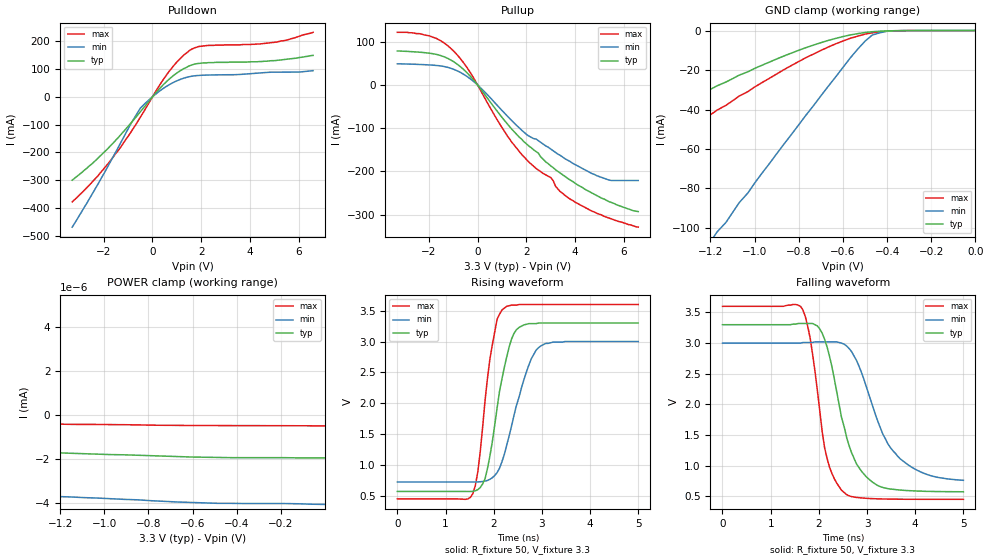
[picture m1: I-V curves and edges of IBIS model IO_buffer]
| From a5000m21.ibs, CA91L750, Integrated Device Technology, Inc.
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|   Model data
[Model]   IO_buffer
Model_type   I/O
Polarity   Non-Inverting
Enable   Active-Low
Vinl =   1.33V
Vinh =   1.74V
C_comp   5.0000pF   4.5000pF   5.5000pF
Rref = 0
Cref = 10pF
Vref = 2.0V
Vmeas = 0
|   |   |\ |   Rref
|   |Driver| \|------o----/\/\/\----o Vref
|   |   | /|   |
|   |   |/ |   === Cref
|   GND
[Temperature Range]   25.0000   80.0000   -40.0000
[Voltage Range]   3.3000V   3.0000V   3.6000V
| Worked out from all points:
|   slope of the pulldown table from 0 to 0.495 V, typ, clamps not added: 10.3 ohm
|   slope of the pullup table from 0 to 0.495 V, typ, clamps not added: 13.2 ohm
|   GND clamp passes 1 mA (typ) near -0.50 V on its own axis
|   POWER clamp passes 1 mA (typ) near -3.79 V on its own axis
|   rising waveform, R_fixture 50, V_fixture 3.3: 20-80 % time 357ps typ, 473ps min, 277ps max; typ from 0.571 V to 3.3 V
|   falling waveform, R_fixture 50, V_fixture 3.3: 20-80 % time 500ps typ, 711ps min, 343ps max; typ from 3.3 V to 0.573 V
[Pulldown]
|   voltage   I(typ)   I(min)   I(max)
-3.3V     -300mA     -469mA     -378mA
-2.5V     -242mA     -353mA     -309mA
-1.8V     -183mA     -245mA     -238mA
-1.3V     -136mA     -164mA     -180mA
-500mV    -54mA      -40.9mA    -73.6mA
500mV     48.4mA     33.5mA     69.2mA
900mV     79mA       53.5mA     115mA
1.3V      102mA      67.4mA     151mA
1.6V      114mA      73.8mA     171mA
1.9V      120mA      76.8mA     181mA
5.1V      131mA      88.7mA     197mA
6.6V      149mA      94.1mA     232mA
[Pullup]
|   voltage   I(typ)   I(min)   I(max)
-3.3V     78.9mA     49.1mA     122mA
-2V       73.7mA     46.5mA     114mA
-1V       54.5mA     36.7mA     79.4mA
-500mV    32mA       22.2mA     45.5mA
-330pV    -132uA     -5.16uA    -63.1uA
1.4V      -102mA     -82.2mA    -132mA
2.1V      -141mA     -118mA     -178mA
3V        -187mA     -148mA     -214mA
3.4V      -204mA     -163mA     -247mA
4V        -227mA     -184mA     -271mA
5.4V      -270mA     -220mA     -308mA
6.6V      -293mA     -221mA     -329mA
[GND_clamp]
|   voltage   I(typ)   I(min)   I(max)
-3.3V     -156mA     -418mA     -194mA
-2.37V    -100mA     -283mA     -129mA
-1.97V    -75.5mA    -223mA     -100mA
-1.17V    -28mA      -102mA     -40.3mA
-1.13V    -26.1mA    -97.2mA    -37.9mA
-1.07V    -22.6mA    -87.2mA    -33.2mA
-1.03V    -20.9mA    -82.2mA    -30.9mA
-767mV    -8.65mA    -42.8mA    -13.7mA
-567mV    -2.25mA    -13.9mA    -3.94mA
-467mV    -611uA     -2.27mA    -1.18mA
-367mV    -101uA     -184uA     -124uA
0V        -112pA     -180pA     -88.4pA
[POWER_clamp]
|   voltage   I(typ)   I(min)   I(max)
-6V       121mA      375mA      132mA
-3.7V     254uA      32.7mA     109nA
-3.64V    59.7uA     23.9mA     4.35nA
-3.58V    21.4uA     15.5mA     216pA
-3.52V    3.68uA     7.79mA     -81.9pA
-3.33V    15.7nA     66.5uA     -133pA
-3.27V    42.2pA     29.3uA     -140pA
-3.21V    -858pA     2.4uA      -148pA
-3.03V    -1.13nA    27.6nA     -171pA
-2.97V    -1.16nA    -1.13nA    -178pA
-2.85V    -1.2nA     -2.77nA    -193pA
-600nV    -1.94nA    -4.06nA    -480pA
[Ramp]
| variable   typ   min   max
dV/dt_r   1.464/0.51n   1.14/0.83n   1.758/0.32n
dV/dt_f   1.23/0.29n   1.23/0.57n   1.23/0.18n
R_load = 50.0000
[Rising Waveform]
R_fixture = 50
V_fixture = 3.3
V_fixture_min = 3.0
V_fixture_max = 3.6
|   Time   V(typ)   V(min)   V(max)
0s        571mV      724mV      450mV
1.57ns    573mV      724mV      541mV
1.67ns    600mV      725mV      888mV
1.82ns    777mV      738mV      2.04V
1.97ns    1.37V      792mV      2.94V
2.07ns    1.92V      876mV      3.36V
2.17ns    2.39V      1.05V      3.51V
2.47ns    3.19V      1.96V      3.59V
2.93ns    3.3V       2.9V       3.6V
5ns       3.3V       3V         3.6V
[Falling Waveform]
R_fixture = 50
V_fixture = 3.3
V_fixture_min = 3.0
V_fixture_max = 3.6
|   Time   V(typ)   V(min)   V(max)
0s        3.3V       3V         3.6V
1.62ns    3.32V      3V         3.6V
1.82ns    3.32V      3.01V      3.08V
2.07ns    3.16V      3.02V      1.55V
2.17ns    2.94V      3.02V      1.12V
2.58ns    1.45V      2.95V      526mV
2.98ns    822mV      2.3V       467mV
3.54ns    614mV      1.24V      453mV
4.14ns    583mV      888mV      450mV
5ns       573mV      760mV      450mV
